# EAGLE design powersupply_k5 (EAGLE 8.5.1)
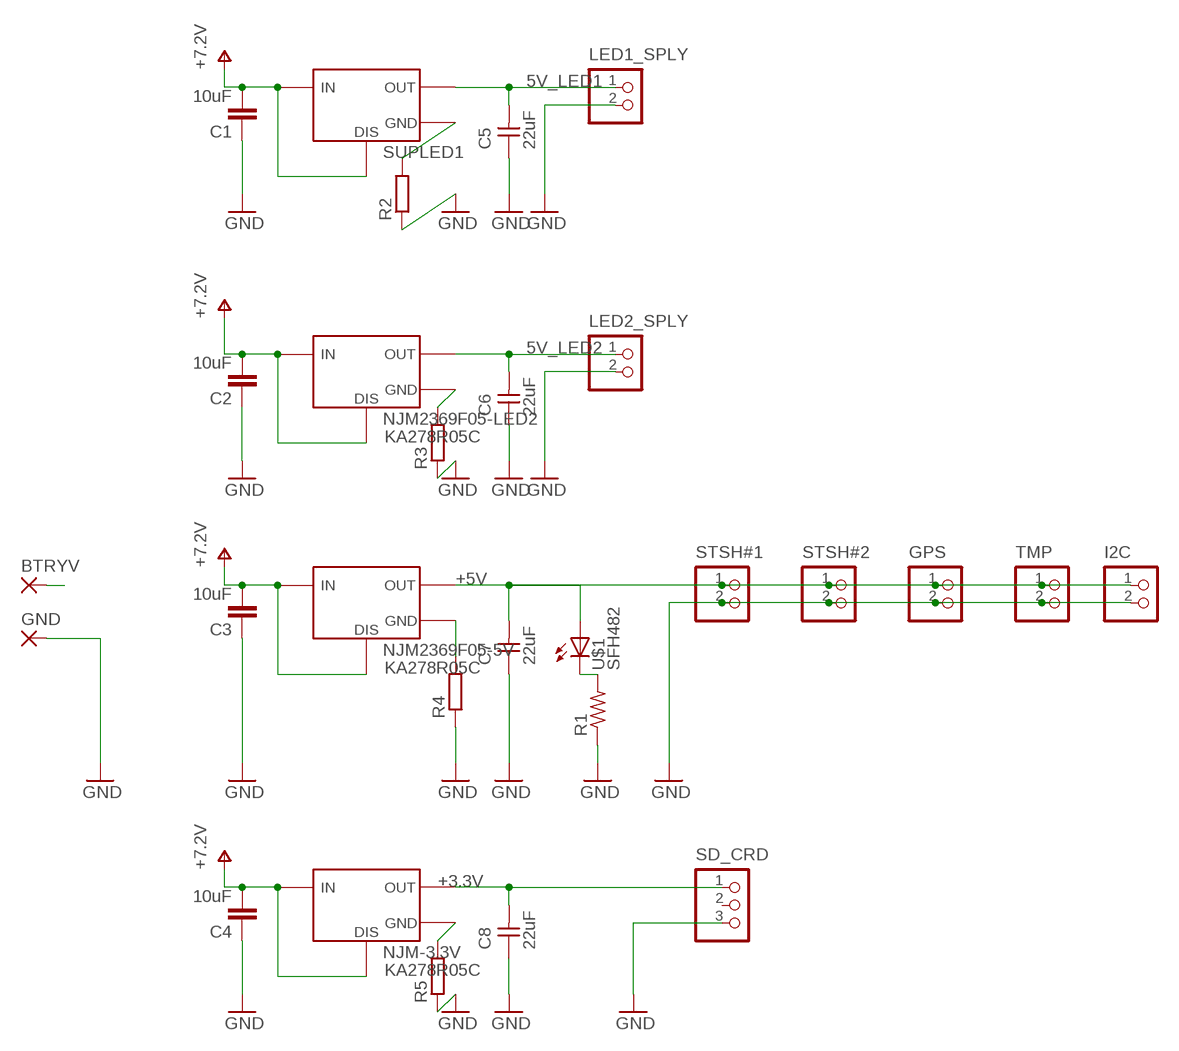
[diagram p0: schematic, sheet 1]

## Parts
BTRYV  3,81/1,1  [3,81/1,1]
C1  10uF  C-EU050-075X075  [C050-075X075]
C2  10uF  C-EU050-075X075  [C050-075X075]
C3  10uF  C-EU050-075X075  [C050-075X075]
C4  10uF  C-EU050-075X075  [C050-075X075]
C5  22uF  CAP-UNPOLARIZEDFAB  [C1206FAB]
C6  22uF  CAP-UNPOLARIZEDFAB  [C1206FAB]
C7  22uF  CAP-UNPOLARIZEDFAB  [C1206FAB]
C8  22uF  CAP-UNPOLARIZEDFAB  [C1206FAB]
GND  3,81/1,1  [3,81/1,1]
GPS  B2B-XH-A  [B2B-XH-A]
I2C  B2B-XH-A  [B2B-XH-A]
LED1_SPLY  B2B-XH-A  [B2B-XH-A]
LED2_SPLY  B2B-XH-A  [B2B-XH-A]
NJM2369F05-5V  KA278R05C  [KA278R05C]
NJM2369F05-LED2  KA278R05C  [KA278R05C]
NJM-3.3V  KA278R05C  [KA278R05C]
R1  RES-US1206FAB  [R1206FAB]
R2  R-EU_0204/7  [0204/7]
R3  R-EU_0204/7  [0204/7]
R4  R-EU_0204/7  [0204/7]
R5  R-EU_0204/7  [0204/7]
SD_CRD  B3B-XH-A  [B3B-XH-A]
STSH#1  B2B-XH-A  [B2B-XH-A]
STSH#2  B2B-XH-A  [B2B-XH-A]
SUPLED1  KA278R05C  [KA278R05C]
TMP  B2B-XH-A  [B2B-XH-A]
U$1  SFH482  [SFH482]

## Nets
5V_LED1: C5.2 LED1_SPLY.1 SUPLED1.VOUT
5V_LED2: C6.2 LED2_SPLY.1 NJM2369F05-LED2.VOUT
+3.3V: C8.2 NJM-3.3V.VOUT SD_CRD.1
+5V: C7.2 GPS.1 I2C.1 NJM2369F05-5V.VOUT STSH#1.1 STSH#2.1 TMP.1 U$1.A
+7.2V: BTRYV.1(P) C1.2 C2.2 C3.2 C4.2 NJM2369F05-5V.VDIS NJM2369F05-5V.VIN NJM2369F05-LED2.VDIS NJM2369F05-LED2.VIN NJM-3.3V.VDIS NJM-3.3V.VIN SUPLED1.VDIS SUPLED1.VIN
GND: C1.1 C2.1 C3.1 C4.1 C5.1 C6.1 C7.1 C8.1 GND.1(P) GPS.2 I2C.2 LED1_SPLY.2 LED2_SPLY.2 NJM2369F05-5V.GND NJM2369F05-LED2.GND NJM-3.3V.GND R1.1 R2.1 R2.2 R3.1 R3.2 R4.1 R4.2 R5.1 R5.2 SD_CRD.3 STSH#1.2 STSH#2.2 SUPLED1.GND TMP.2
N$1: R1.2 U$1.K(C)
Unconnected: SD_CRD.2

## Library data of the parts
BTRYV GND = wirepad:3,81/1,1: THROUGH-HOLE PAD
C1-C4 = rcl:C-EU: CAPACITOR, European symbol; SPICEPREFIX: C
C5-C8 = fab:CAP-UNPOLARIZED
GPS I2C LED1_SPLY LED2_SPLY STSH#1 STSH#2 TMP = jst-xh:B2B-XH-A: Wire-to-Board 2.5mm pitch top mount connector
NJM2369F05-5V NJM2369F05-LED2 NJM-3.3V SUPLED1 = v-reg-fairchild:KA278R05C
R1 = fab:RES-US: Resistor (US Symbol)
R2-R5 = rcl:R-EU_: RESISTOR, European symbol; SPICEPREFIX: R
SD_CRD = jst-xh:B3B-XH-A: Wire-to-Board 2.5mm pitch top mount connector Source: http://www.jst-mfg.com/product/pdf/jpn/XH.pdf http://www.jst-mfg.com/product/detail.php?series=277
U$1 = led:SFH482: IR LED

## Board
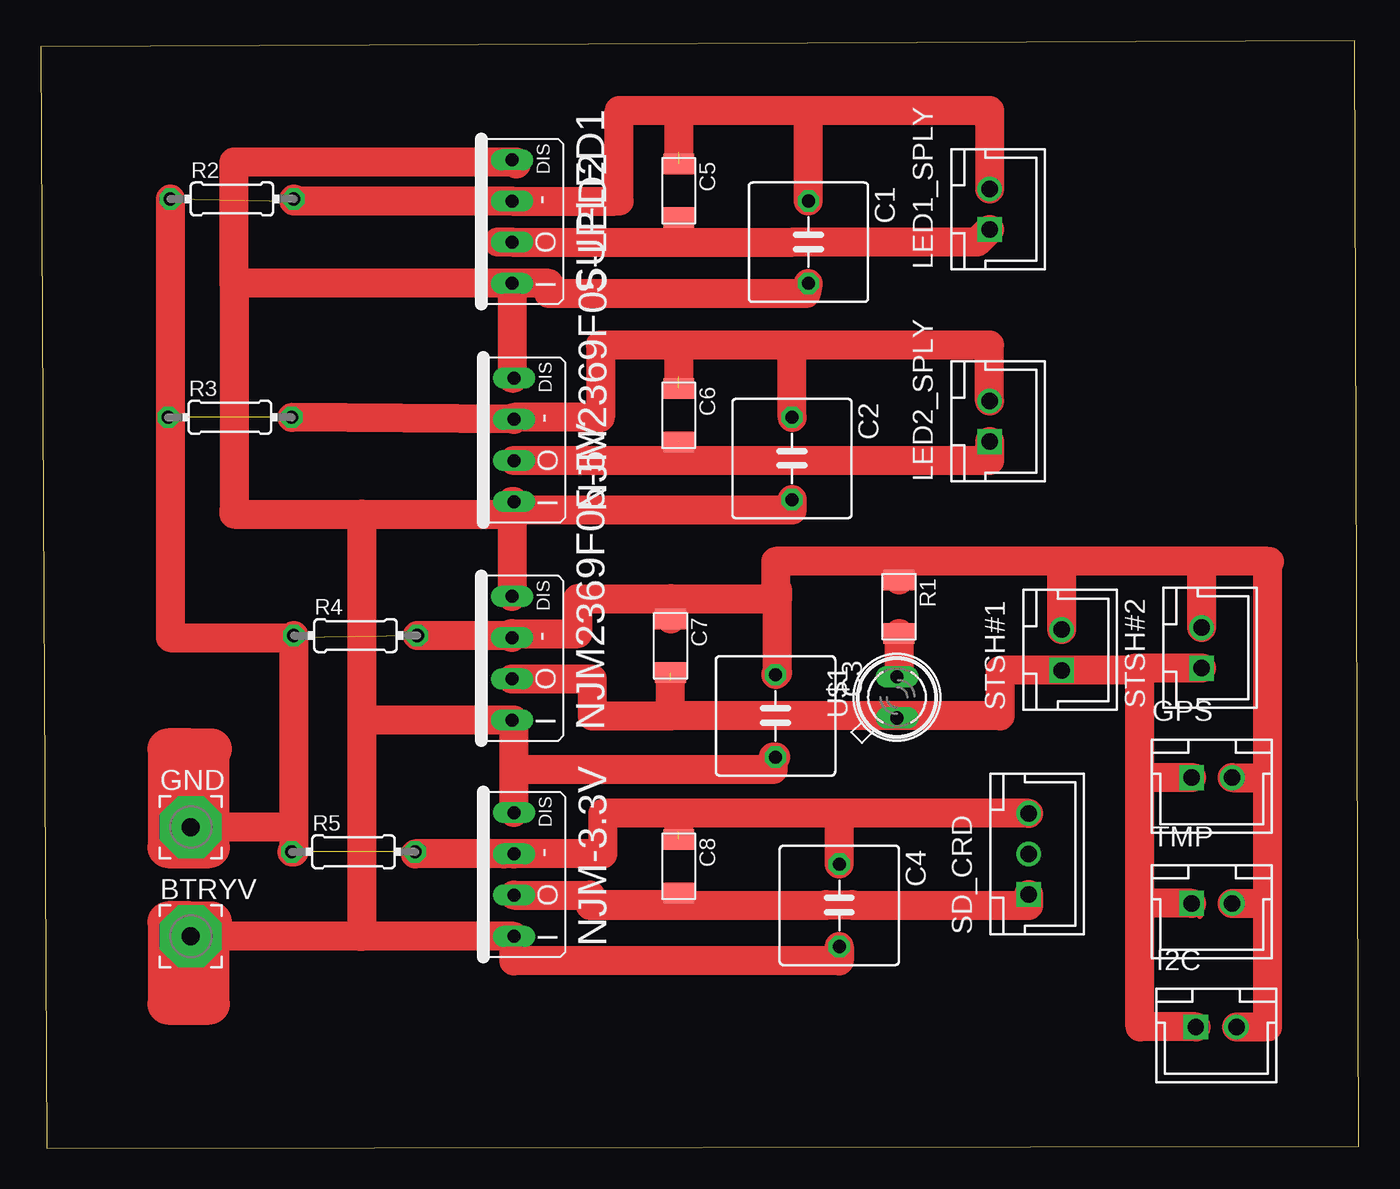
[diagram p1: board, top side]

Size 81.33 x 68.32 mm. Coordinates in mm from the lower left corner, seen from the top.
Outline: 0.38,0 81.33,0.13 81.08,68.32 0,67.94 0.38,0
Copper layers (1*16): Top 0.035mm / dielectric 1.5mm / Bottom 0.035mm
Design rules "default *": minimum track width 6mil, minimum drill 0.35mm, track to track 0.4mm, track to pad 0.4mm, pad to pad 0.4mm, via to via 0.4mm, smd to smd 0.4mm, copper to edge 40mil, drill to drill 6mil, minimum pad ring 10mil, minimum via ring 8mil, stop-mask expansion 4mil, vias tented up to drill 0mil, thermal gap 10mil

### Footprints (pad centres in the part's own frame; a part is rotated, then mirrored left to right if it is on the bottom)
3,81/1,1 = drill 1.118 pad 3.81 octagon: 1 0,0
C050-075X075 = drill 0.813 octagon: 1 -2.54,0; 2 2.54,0
C1206FAB = smd 1.27 x 1.905: 1 -1.651,0; 2 1.651,0
B2B-XH-A = drill 1.016 square: 1 -1.25,0 | drill 1.016: 2 1.25,0
KA278R05C = drill 0.8 long: GND 1.27,1.27; VDIS 3.81,1.27; VIN -3.81,1.27; VOUT -1.27,1.27
R1206FAB = smd 1.27 x 1.905: 1 -1.651,0; 2 1.651,0
0204/7 = drill 0.813 octagon: 1 -3.81,0; 2 3.81,0
B3B-XH-A = drill 1.016 square: 1 -2.5,0 | drill 1.016: 2 0,0; 3 2.5,0
SFH482 = drill 0.813 long: A -1.27,0; K 1.27,0

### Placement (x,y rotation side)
BTRYV  9.27,13.08 0 top
C1  47.37,55.88 270 top
C2  46.35,42.55 270 top
C3  45.34,26.67 270 top
C4  49.28,14.99 270 top
C5  39.37,59.05 270 top
C6  39.37,45.21 270 top
C7  38.86,30.99 270 top
C8  39.37,17.4 270 top
GND  9.27,19.81 0 top
GPS  72.26,22.86 0 top
I2C  72.52,7.49 0 top
LED1_SPLY  58.55,57.91 90 top
LED2_SPLY  58.55,44.83 90 top
NJM2369F05-5V  30.35,30.23 90 top
NJM2369F05-LED2  30.48,43.69 90 top
NJM-3.3V  30.48,16.89 90 top
R1  52.96,33.4 270 top
R2  11.81,58.55 0 top
R3  11.68,45.09 0 top
R4  19.43,31.62 0 top
R5  19.3,18.29 0 top
SD_CRD  60.96,18.16 90 top
STSH#1  62.99,30.73 90 top
STSH#2  71.63,30.86 90 top
SUPLED1  30.35,57.15 90 top
TMP  72.26,15.11 0 top
U$1  52.83,27.81 90 top

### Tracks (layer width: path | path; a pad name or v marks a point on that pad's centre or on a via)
5V_LED1
  Top 0.254: C5.2 39.37,55.88 39.24,55.88
  Top 1.778: 28.19,55.88 SUPLED1.VOUT 39.24,55.88 46.42,55.88 46.44,55.91 57.79,55.91 LED1_SPLY.1
5V_LED2  (1 unrouted)
  Top 0.406: 39.37,43.58 C6.2 | 35.18,42.04 29.21,42.04 | 28.83,42.04 29.21,42.04 | 29.21,42.04 NJM2369F05-LED2.VOUT
  Top 0.508: C6.2 39.12,43.56 39.12,42.42
  Top 1.778: LED2_SPLY.1 58.55,42.42 39.12,42.42 NJM2369F05-LED2.VOUT
+3.3V
  Top 0.406: SD_CRD.1 39.5,15.03 C8.2 29.84,15.75 NJM-3.3V.VOUT
  Top 1.778: NJM-3.3V.VOUT 33.91,15.62 33.91,14.99 48.42,14.99 48.47,15.03 50.08,15.03 50.13,14.99 60.96,14.99 SD_CRD.1
+5V  (1 unrouted)
  Top 0.406: 38.86,27.05 38.86,26.54 U$1.A 52.83,26.67 59.18,26.67 | 62.99,29.59 STSH#1.1 | STSH#1.1 67.56,29.48 | 67.82,29.48 71.63,29.48 STSH#2.1 | 71.39,23.49 GPS.1 | 71.52,14.35 TMP.1 | STSH#1.1 59.56,29.48
  Top 1.778: I2C.1 67.82,7.49 67.82,15.11 | 67.82,15.11 67.82,22.86 | 67.82,22.86 67.82,29.48 67.56,29.48 | 67.56,29.48 59.56,29.48 59.18,29.48 59.18,26.67 38.86,26.67 | 38.86,26.67 38.86,27.05 38.86,28.83 | NJM2369F05-5V.VOUT 34.04,28.96 34.04,26.67 38.86,26.67 | STSH#2.1 67.56,29.61 67.56,29.48 | GPS.1 67.82,22.86 | TMP.1 67.82,15.11
+7.2V
  Top 0.406: 29.08,53.21 SUPLED1.VIN 28.45,53.34 11.94,53.34 | 11.94,53.34 11.94,39.37 11.94,39.12 11.94,38.48 | 29.21,40.01 NJM2369F05-LED2.VIN 39.5,39.88 | 29.97,34.16 NJM2369F05-5V.VDIS 29.08,39.37 28.83,39.37 | NJM2369F05-LED2.VDIS 29.21,50.17 | SUPLED1.VDIS 29.34,60.71 12.19,60.83 12.07,60.83 12.07,53.47 11.94,53.34 | 19.69,13.08 20.07,13.08 20.07,26.54 NJM2369F05-5V.VIN 29.21,26.42 | 8.64,13.08 BTRYV.1 | 29.21,23.62 29.21,23.37
  Top 1.778: C1.2 47.24,52.71 31.37,52.71 31.37,53.34 28.45,53.34 | C2.2 46.35,39.37 28.83,39.37 28.83,39.12 19.81,39.12 | 11.94,53.34 SUPLED1.VIN 29.08,47.5 NJM2369F05-LED2.VDIS | 12.07,53.47 11.94,53.47 | 11.94,53.47 11.94,39.37 | 11.94,39.12 19.81,39.12 | 19.81,39.12 19.81,26.42 | 19.81,26.42 19.81,13.08 | 19.81,13.08 19.69,13.08 BTRYV.1 | 29.21,23.62 29.21,26.42 | C3.2 45.21,24.13 45.21,23.37 29.21,23.37 NJM-3.3V.VDIS | NJM2369F05-5V.VIN 19.81,26.42 | C4.2 49.28,11.56 29.21,11.56 NJM-3.3V.VIN 19.81,13.08 | NJM2369F05-LED2.VIN 29.08,39.88 NJM2369F05-5V.VDIS | 11.94,53.47 11.94,60.83 12.19,60.83 29.34,60.83 29.34,60.71
  Top 2.54: BTRYV.1 9.27,13.97 | 9.27,13.97 10.54,13.97 | 9.27,13.97 7.87,13.97 7.87,8.89 10.41,8.89 10.41,13.84
GND  (12 unrouted)
  Top 0.406: 34.67,18.16 NJM-3.3V.GND 28.58,18.16 23.11,18.16 R5.2 | R2.1 8,45.09 R3.1 8,31.5 R4.1 15.62,31.37 15.62,18.29 | R5.1 15.49,19.81 | 55.12,21.21 60.96,21.21 SD_CRD.3 | 73.77,23.49 GPS.2 | 71.63,32.24 STSH#2.2 | 62.99,32.11 STSH#1.2 | C7.1 38.86,32.51 | R1.1 52.96,34.54 | 39.37,64.01 39.37,63.75 | 46.99,64.01 39.5,64.01 39.37,64.01 | C2.1 46.35,46.86 | LED2_SPLY.2 58.55,46.23 | 58.55,64.01 58.93,64.01 | 47.37,64.01 46.99,64.01 | 46.99,64.01 47.37,63.99 | 35.43,58.42 35.69,58.42 | 35.56,64.01 35.69,64.01 39.37,64.01
  Top 1.778: SUPLED1.GND 35.43,58.42 | 35.69,58.42 35.69,64.01 39.5,64.01 47.37,64.01 | 47.37,64.01 58.55,64.01 LED1_SPLY.2 | C1.1 47.37,64.01 | 39.37,63.75 39.37,61.47 | SUPLED1.GND | LED2_SPLY.2 58.55,49.53 46.35,49.53 | 46.35,49.53 39.37,49.53 | 39.37,49.53 39.37,47.62 | C2.1 46.35,49.53 | 39.37,49.53 34.54,49.53 34.54,45.09 29.21,45.09 NJM2369F05-LED2.GND R3.2 | R2.2 15.62,58.42 SUPLED1.GND | R2.1 8,31.5 | 8,31.5 | 8,31.5 15.62,31.5 15.62,31.37 | R4.1 15.62,18.29 R5.1 | 15.49,19.81 GND.1 | I2C.2 75.69,7.49 75.69,15.11 | 75.69,15.11 75.69,22.86 | 75.69,22.86 75.69,36.2 | 75.69,36.2 75.82,36.2 | 75.69,36.2 71.63,36.2 | 71.63,36.2 62.99,36.2 | 62.99,36.2 52.96,36.2 | 52.96,36.2 45.34,36.2 45.34,34.42 45.47,34.42 45.47,33.91 | 38.86,33.91 45.47,33.91 | C3.1 45.47,29.34 45.47,33.91 | STSH#1.2 62.99,36.2 | STSH#2.2 71.63,36.2 | 52.96,36.2 R1.1 | C7.1 38.86,33.91 | 38.86,33.91 33.15,33.91 33.15,31.75 29.08,31.75 NJM2369F05-5V.GND 29.08,31.62 R4.2 | GPS.2 75.69,22.86 | TMP.2 75.69,15.11 | SD_CRD.3 49.28,20.66 | 49.28,20.66 39.37,20.66 | 39.37,20.66 34.67,20.66 34.67,18.16 28.58,18.16 | NJM-3.3V.GND 23.11,18.16 | C4.1 49.28,20.66 | 39.37,20.66 39.37,19.56
  Top 2.54: GND.1 9.27,24.64 | 9.27,24.64 10.16,24.64 | 9.27,24.64 7.87,24.64 7.87,18.54 10.41,18.54 10.41,24.64 10.54,24.64
N$1
  Top 0.406: 52.96,29.72 52.96,29.08 U$1.K
  Top 1.778: R1.2 52.96,29.72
